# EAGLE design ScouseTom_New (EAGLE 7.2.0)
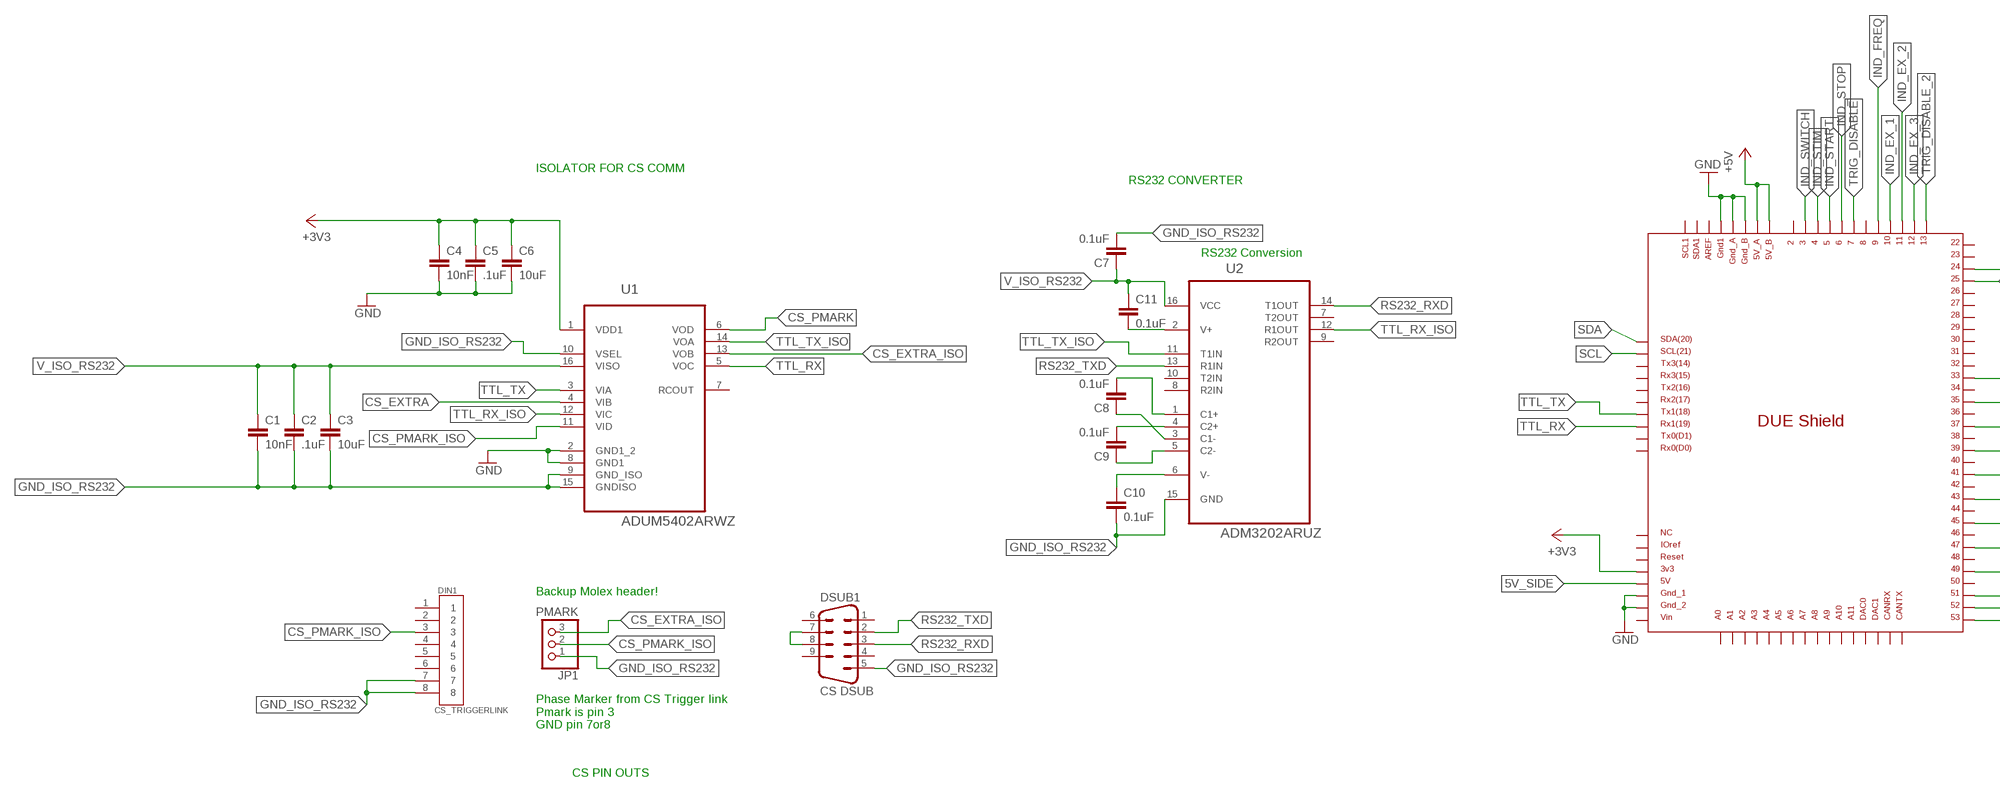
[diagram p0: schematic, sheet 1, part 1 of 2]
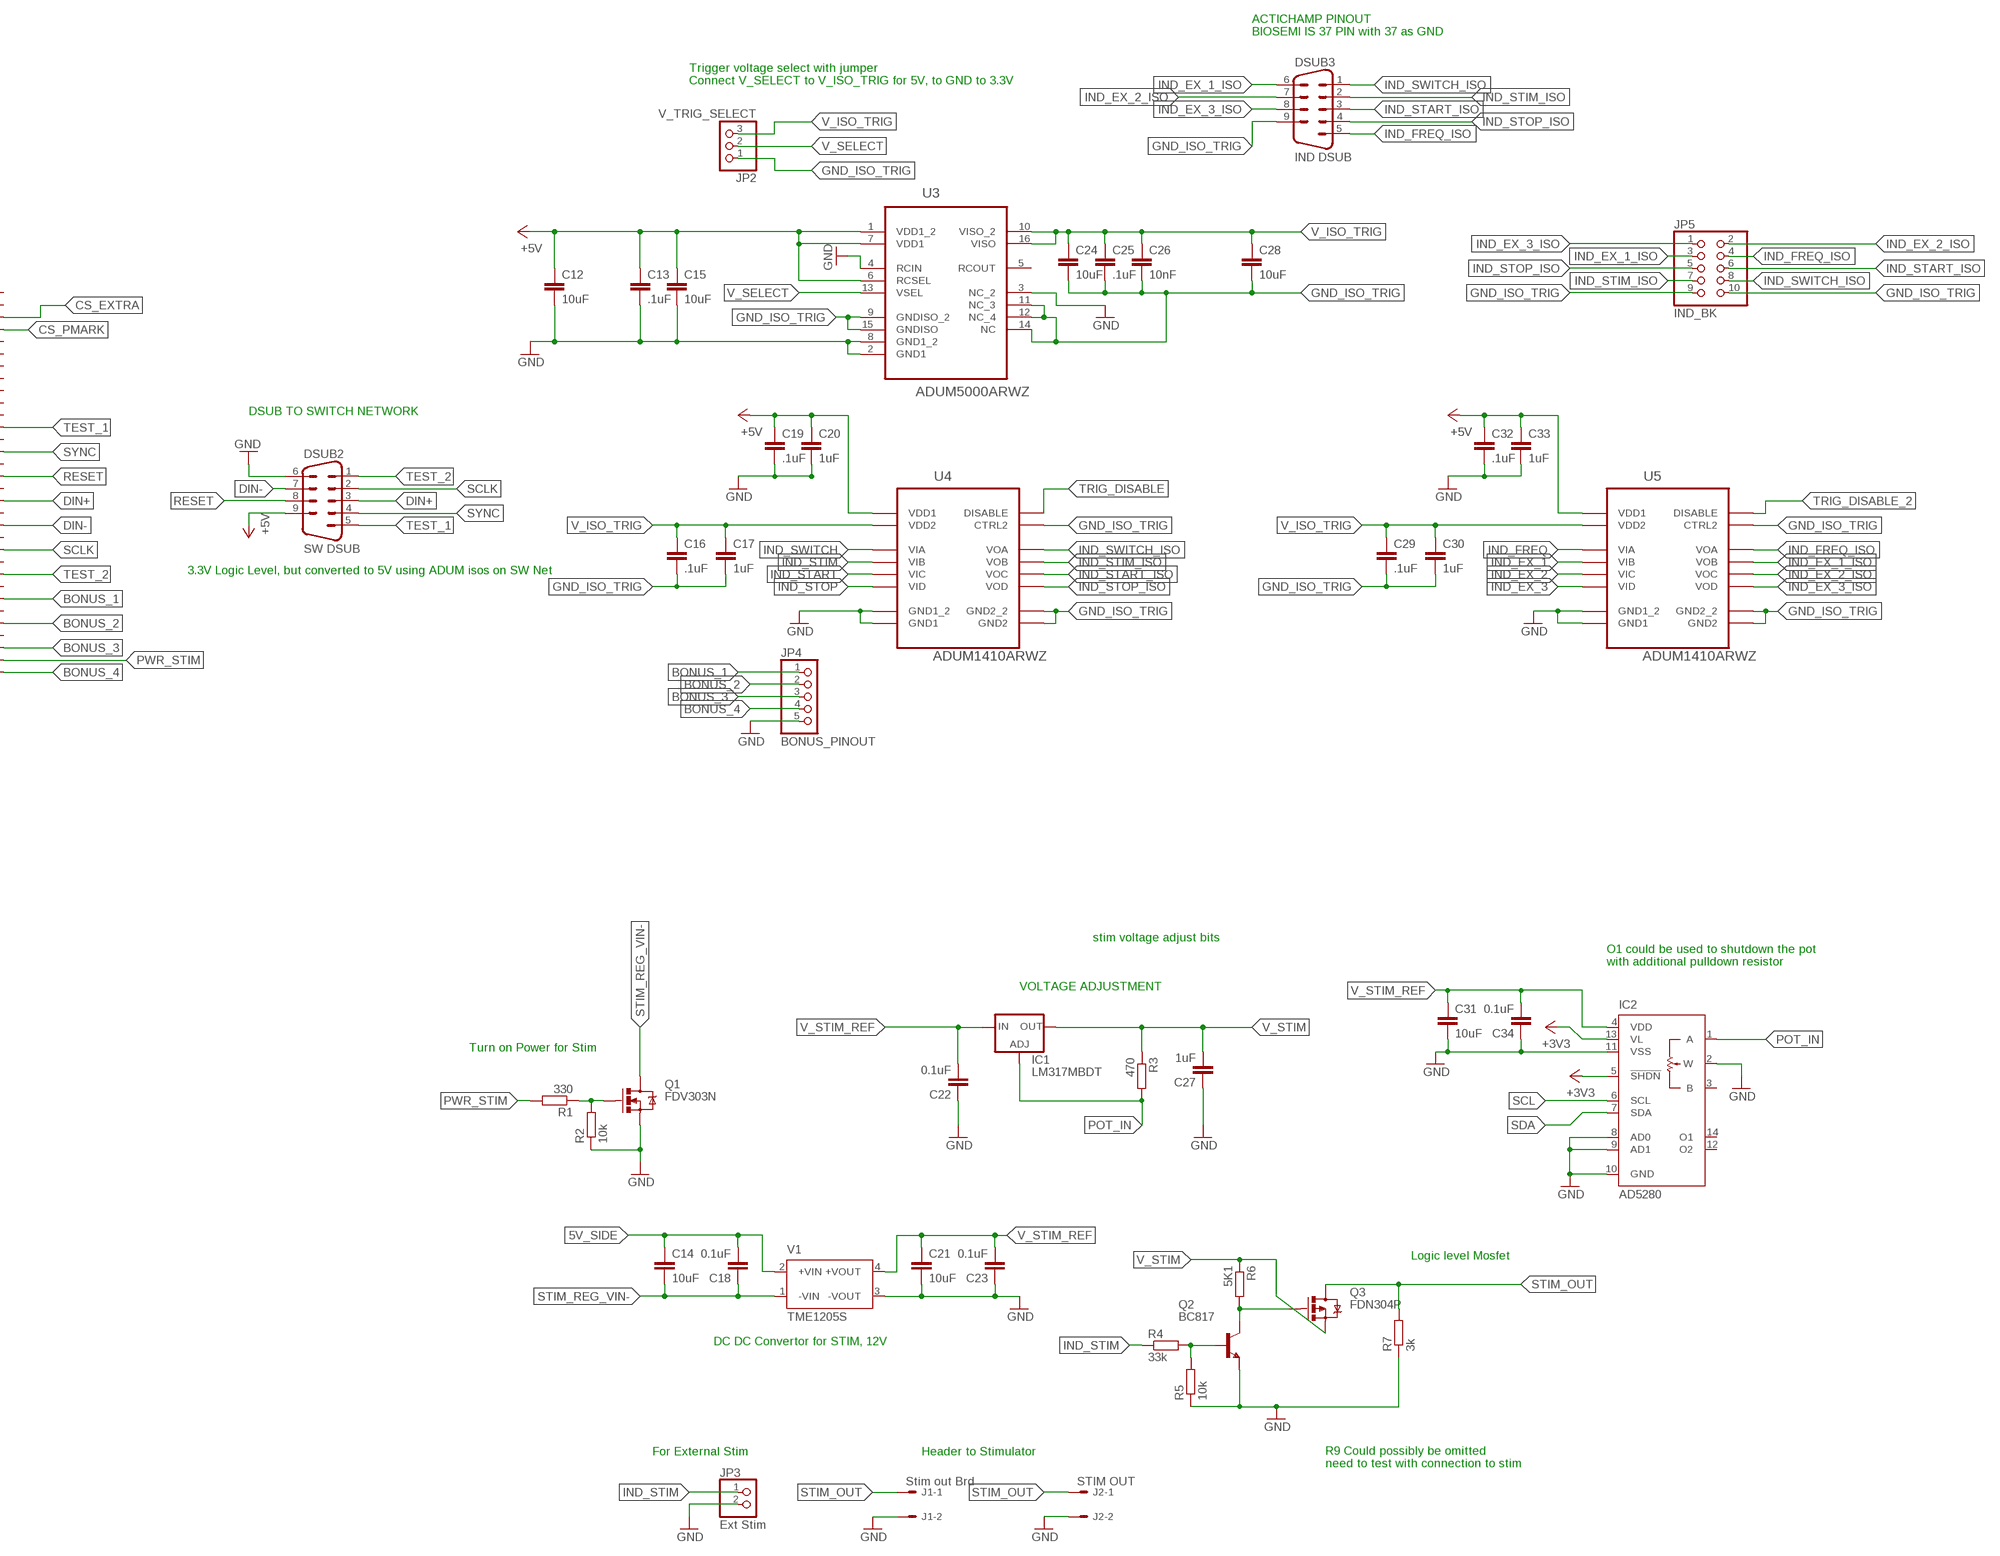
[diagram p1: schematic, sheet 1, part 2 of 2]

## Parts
ARD1  DUE(NOMID)  [DUE(NOMID)]
C1  10nF  C-EUC0805  [C0805]
C2  .1uF  C-EUC0805  [C0805]
C3  10uF  C-EUC0805  [C0805]
C4  10nF  C-EUC0805  [C0805]
C5  .1uF  C-EUC0805  [C0805]
C6  10uF  C-EUC0805  [C0805]
C7  0.1uF  C-EUC0805  [C0805]
C8  0.1uF  C-EUC0805  [C0805]
C9  0.1uF  C-EUC0805  [C0805]
C10  0.1uF  C-EUC0805  [C0805]
C11  0.1uF  C-EUC0805  [C0805]
C12  10uF  C-EUC0805  [C0805]
C13  .1uF  C-EUC0805  [C0805]
C14  10uF  C-EUC0805  [C0805]
C15  10uF  C-EUC0805  [C0805]
C16  .1uF  C-EUC0805  [C0805]
C17  1uF  C-EUC0805  [C0805]
C18  0.1uF  C-EUC0805  [C0805]
C19  .1uF  C-EUC0805  [C0805]
C20  1uF  C-EUC0805  [C0805]
C21  10uF  C-EUC0805  [C0805]
C22  0.1uF  C-EUC0805  [C0805]
C23  0.1uF  C-EUC0805  [C0805]
C24  10uF  C-EUC0805  [C0805]
C25  .1uF  C-EUC0805  [C0805]
C26  10nF  C-EUC0805  [C0805]
C27  1uF  C-EUC0805  [C0805]
C28  10uF  C-EUC0805  [C0805]
C29  .1uF  C-EUC0805  [C0805]
C30  1uF  C-EUC0805  [C0805]
C31  10uF  C-EUC0805  [C0805]
C32  .1uF  C-EUC0805  [C0805]
C33  1uF  C-EUC0805  [C0805]
C34  0.1uF  C-EUC0805  [C0805]
DIN1  CS_TRIGGERLINK  DIN8  [DIN8]
DSUB1  CS DSUB  DSUB9RA  [DSUB9]
DSUB2  SW DSUB  DSUB9RA  [DSUB9]
DSUB3  IND DSUB  DSUB9RA  [DSUB9]
IC1  LM317MBDT  [DPACK]
IC2  AD5280  [TSSOP14]
J1  Stim out Brd  22-27-2021-02  [6410-02]
J2  STIM OUT  22-05-7028-02  [7395-02]
JP1  PMARK  PINHD-1X3  [1X03]
JP2  V_TRIG_SELECT  PINHD-1X3  [1X03]
JP3  Ext Stim  PINHD-1X2  [1X02]
JP4  BONUS_PINOUT  PINHD-1X5  [1X05]
JP5  IND_BK  PINHD-2X5  [2X05]
Q1  FDV303N  MOSFET-NCHANNEL2N7002PW  [SOT323]
Q2  BC817  BC817-40SMD  [SOT23-BEC]
Q3  FDN304P  MOSFET-PCHANNEL  [SOT23-3]
R1  330  R-EU_R0805  [R0805]
R2  10k  R-EU_R0805  [R0805]
R3  470  R-EU_R0805  [R0805]
R4  33k  R-EU_R0805  [R0805]
R5  10k  R-EU_R0805  [R0805]
R6  5K1  R-EU_R0805  [R0805]
R7  3k  R-EU_R0805  [R0805]
U1  ADUM5402ARWZ  [SOIC127P1032X265-16N]
U2  ADM3202ARUZ  [SOP65P640X120-16N]
U3  ADUM5000ARWZ  [SOIC127P1032X265-16N]
U4  ADUM1410ARWZ  [SOIC127P1032X265-16N]
U5  ADUM1410ARWZ  [SOIC127P1032X265-16N]
V1  TME1205S  [TME]

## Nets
5V_SIDE: ARD1.5V C14.1 C18.2 V1.2(+VIN)
+3V3: ARD1.3V3 C4.1 C5.1 C6.1 IC2.5(!SHDN) IC2.13(VL) U1.1(VDD1)
+5V: ARD1.5V_A ARD1.5V_B C12.1 C13.1 C15.1 C19.1 C20.1 C32.1 C33.1 DSUB2.9 U3.1(VDD1_2) U3.6(RCSEL) U3.7(VDD1) U4.1(VDD1) U5.1(VDD1)
BONUS_1: ARD1.47 JP4.1
BONUS_2: ARD1.49 JP4.2
BONUS_3: ARD1.51 JP4.3
BONUS_4: ARD1.53 JP4.4
CS_EXTRA: ARD1.24 U1.4(VIB)
CS_EXTRA_ISO: JP1.3 U1.13(VOB)
CS_PMARK: ARD1.25 U1.6(VOD)
CS_PMARK_ISO: DIN1.3 JP1.2 U1.11(VID)
DIN+: ARD1.39 DSUB2.3
DIN-: ARD1.41 DSUB2.7
GND: ARD1.GND1 ARD1.GND_1 ARD1.GND_2 ARD1.GND_A ARD1.GND_B C4.2 C5.2 C6.2 C12.2 C13.2 C15.2 C19.2 C20.2 C21.2 C22.1 C23.1 C27.1 C31.2 C32.2 C33.2 C34.1 DSUB2.6 IC2.2(W) IC2.8(AD0) IC2.9(AD1) IC2.10(GND) IC2.11(VSS) J1.2 J2.2 JP3.2 JP4.5 Q1.2(S) Q2.E R2.1 R5.1 R7.1 U1.2(GND1_2) U1.8(GND1) U3.2(GND1) U3.3(NC_2) U3.4(RCIN) U3.8(GND1_2) U4.2(GND1_2) U4.8(GND1) U5.2(GND1_2) U5.8(GND1) V1.3(-VOUT)
GND_ISO_RS232: C1.2 C2.2 C3.2 C7.2 C10.2 DIN1.7 DIN1.8 DSUB1.5 JP1.1 U1.9(GND_ISO) U1.10(VSEL) U1.15(GNDISO) U2.15(GND)
GND_ISO_TRIG: C16.2 C17.2 C24.2 C25.2 C26.2 C28.2 C29.2 C30.2 DSUB3.9 JP2.1 JP5.9 JP5.10 U3.9(GNDISO_2) U3.11(NC_3) U3.12(NC_4) U3.14(NC) U3.15(GNDISO) U4.9(GND2_2) U4.10(CTRL2) U4.15(GND2) U5.9(GND2_2) U5.10(CTRL2) U5.15(GND2)
IND_EX_1: ARD1.10 U5.4(VIB)
IND_EX_1_ISO: DSUB3.6 JP5.3 U5.13(VOB)
IND_EX_2: ARD1.11 U5.5(VIC)
IND_EX_2_ISO: DSUB3.7 JP5.2 U5.12(VOC)
IND_EX_3: ARD1.12 U5.6(VID)
IND_EX_3_ISO: DSUB3.8 JP5.1 U5.11(VOD)
IND_FREQ: ARD1.9 U5.3(VIA)
IND_FREQ_ISO: DSUB3.5 JP5.4 U5.14(VOA)
IND_START: ARD1.5 U4.5(VIC)
IND_START_ISO: DSUB3.3 JP5.6 U4.12(VOC)
IND_STIM: ARD1.4 JP3.1 R4.1 U4.4(VIB)
IND_STIM_ISO: DSUB3.2 JP5.7 U4.13(VOB)
IND_STOP: ARD1.6 U4.6(VID)
IND_STOP_ISO: DSUB3.4 JP5.5 U4.11(VOD)
IND_SWITCH: ARD1.3 U4.3(VIA)
IND_SWITCH_ISO: DSUB3.1 JP5.8 U4.14(VOA)
N$1: Q2.B R4.2 R5.2
N$3: Q2.C Q3.1(G) R6.2
N$4: DSUB1.7 DSUB1.8
N$5: Q1.1(G) R1.1 R2.2
N$22: C8.2 U2.1(C1+)
N$23: C8.1 U2.3(C1-)
N$24: C9.2 U2.4(C2+)
N$25: C9.1 U2.5(C2-)
N$26: C11.2 U2.2(V+)
N$27: C10.1 U2.6(V-)
POT_IN: IC1.1(ADJ) IC2.1(A) R3.2
PWR_STIM: ARD1.52 R1.2
RESET: ARD1.37 DSUB2.8
RS232_RXD: DSUB1.3 U2.14(T1OUT)
RS232_TXD: DSUB1.2 U2.13(R1IN)
SCL: ARD1.SCL IC2.6(SCL)
SCLK: ARD1.43 DSUB2.2
SDA: ARD1.SDA IC2.7(SDA)
STIM_OUT: J1.1 J2.1 Q3.3(D) R7.2
STIM_REG_VIN-: C14.2 C18.1 Q1.3(D) V1.1(-VIN)
SYNC: ARD1.35 DSUB2.4
TEST_1: ARD1.33 DSUB2.5
TEST_2: ARD1.45 DSUB2.1
TRIG_DISABLE: ARD1.7 U4.7(DISABLE)
TRIG_DISABLE_2: ARD1.13 U5.7(DISABLE)
TTL_RX: ARD1.RX1 U1.5(VOC)
TTL_RX_ISO: U1.12(VIC) U2.12(R1OUT)
TTL_TX: ARD1.TX1 U1.3(VIA)
TTL_TX_ISO: U1.14(VOA) U2.11(T1IN)
V_ISO_RS232: C1.1 C2.1 C3.1 C7.1 C11.1 U1.16(VISO) U2.16(VCC)
V_ISO_TRIG: C16.1 C17.1 C24.1 C25.1 C26.1 C28.1 C29.1 C30.1 JP2.3 U3.10(VISO_2) U3.16(VISO) U4.16(VDD2) U5.16(VDD2)
V_SELECT: JP2.2 U3.13(VSEL)
V_STIM: C27.2 IC1.4(OUT) Q3.2(S) R3.1 R6.1
V_STIM_REF: C21.1 C22.2 C23.2 C31.1 C34.2 IC1.3(IN) IC2.4(VDD) V1.4(+VOUT)
Unconnected: ARD1.2 ARD1.8 ARD1.22 ARD1.23 ARD1.26 ARD1.27 ARD1.28 ARD1.29 ARD1.30 ARD1.31 ARD1.32 ARD1.34 ARD1.36 ARD1.38 ARD1.40 ARD1.42 ARD1.44 ARD1.46 ARD1.48 ARD1.50 ARD1.A0 ARD1.A1 ARD1.A2 ARD1.A3 ARD1.A4 ARD1.A5 ARD1.A6 ARD1.A7 ARD1.A8 ARD1.A9 ARD1.A10 ARD1.A11 ARD1.AREF ARD1.CANRX ARD1.CANTX ARD1.DAC0 ARD1.DAC1 ARD1.IOREF ARD1.NC ARD1.RESET ARD1.RX0 ARD1.RX2 ARD1.RX3 ARD1.SCL1 ARD1.SDA1 ARD1.TX0 ARD1.TX2 ARD1.TX3 ARD1.VIN DIN1.1 DIN1.2 DIN1.4 DIN1.5 DIN1.6 DSUB1.1 DSUB1.4 DSUB1.6 DSUB1.9 IC2.3(B) IC2.12(O2) IC2.14(O1) U1.7(RCOUT) U2.7(T2OUT) U2.8(R2IN) U2.9(R2OUT) U2.10(T2IN) U3.5(RCOUT)

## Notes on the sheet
- ACTICHAMP PINOUT
  BIOSEMI IS 37 PIN with 37 as GND
- Trigger voltage select with jumper
  Connect V_SELECT to V_ISO_TRIG for 5V, to GND to 3.3V
- ISOLATOR FOR CS COMM
- RS232 CONVERTER
- RS232 Conversion
- DSUB TO SWITCH NETWORK
- 3.3V Logic Level, but converted to 5V using ADUM isos on SW Net
- Backup Molex header!
- Phase Marker from CS Trigger link
  Pmark is pin 3
  GND pin 7or8
- CS PIN OUTS
- stim voltage adjust bits
- O1 could be used to shutdown the pot
  with additional pulldown resistor
- VOLTAGE ADJUSTMENT
- Turn on Power for Stim
- Logic level Mosfet
- DC DC Convertor for STIM, 12V
- For External Stim | Header to Stimulator
- R9 Could possibly be omitted
  need to test with connection to stim

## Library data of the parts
ARD1 = DUElib130425_JAMES:DUE(NOMID)
C1-C34 = resistor:C-EU: CAPACITOR, European symbol
DIN1 = mini din 8 james:DIN8
DSUB1-DSUB3 = DSUBJAMES:DSUB9RA
IC1 = v-reg:LM317?*: 500 mA Adjustable Output Positive Voltage Regulator Source: http://www.onsemi.co.jp .. LM317M-D.PDF
IC2 = analog-devices:AD5280: Single +15 V/±5 V, 256-Position, I2C-Compatible Digital Potentiometer Source: http://www.analog.com/static/imported-files/data_sheets/AD5280_5282.pdf; MF: ALTERA CORPORATION; MPN: AD5280BRUZ20; OC_FARNELL: 1464325; OC_NEWARK: 59K3840
J1 = con-molex:22-?-02: CONNECTOR; OC_FARNELL: unknown; OC_NEWARK: unknown
J2 = con-molex:22-?-02: CONNECTOR; OC_FARNELL: 9731601; OC_NEWARK: unknown
JP1 JP2 = pinhead:PINHD-1X3: PIN HEADER
JP3 = pinhead:PINHD-1X2: PIN HEADER
JP4 = pinhead:PINHD-1X5: PIN HEADER
JP5 = pinhead:PINHD-2X5: PIN HEADER
Q1 = SparkFun-DiscreteSemi:MOSFET-NCHANNEL: Common NMOSFET Parts MFG P/NStore IDProd ID FDD8780TRANS-09984 SI7820DNTRANS-11055 FDS6630AIC-08089 2N7002PWTRANS-11151 FQP30N06L COM-10213TRANS-10060 BSS123LT1GTRANS-08345 BSS138TRANS-00830 BS170 2N7000; PROD_ID: TRANS-11151
Q2 = transistor-npn:BC817*: NPN Transistor
Q3 = SparkFun-DiscreteSemi:MOSFET-PCHANNEL: Generic PMOSFET IRLML2244 - TRANS-11153 (SOT-23 -20V -4.3A) (1.Gate 2.Source 3.Drain) FQP27P06 - COM-10349 (TO-220 -60V -27A) (1.Gate 2.Source 3.Drain); PROD_ID: TRANS-08285
R1-R7 = resistor:R-EU_: RESISTOR, European symbol
U1 = Analog Devices_By_element14_Batch_1:ADUM5402ARWZ: Quad-Channel Isolators with Integrated DC-to-DC Converter; MPN: ADUM5402ARWZ; OC_FARNELL: 1838922; OC_NEWARK: 11N8824; PACKAGE: SOIC-16; SUPPLIER: Analog Devices
U2 = Analog Devices_By_element14_Batch_1:ADM3202ARUZ: Low Power, 3.3 V, RS-232 Line Drivers/Receivers; MPN: ADM3202ARUZ; OC_FARNELL: 9425586; OC_NEWARK: 59K2064; PACKAGE: TSSOP-16; SUPPLIER: Analog Devices
U3 = Analog Devices_By_element14_Batch_1:ADUM5000ARWZ: 2.5 kV, Isolated DC-to-DC Converter; MPN: ADUM5000ARWZ; OC_FARNELL: 1701256; OC_NEWARK: 19P8235; PACKAGE: SOIC-16; SUPPLIER: Analog Devices
U4 U5 = ADI-Phase-2:ADUM1410ARWZ: ISOLATOR, DGTL, 4CHAN; MPN: ADUM1410ARWZ; OC_FARNELL: 2067770; OC_NEWARK: 73T8174; PACKAGE: 16-Lead SOIC_W; SUPPLIER: Analog Devices
V1 = traco-electronic:TME?*: DC/DC Converter TME Series 1 Watt Source: www.tracopower.com .. tme.pdf; MPN: TME 1205S; OC_FARNELL: 1007542; OC_NEWARK: 51R5325

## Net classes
1 power: width 0.61 mm, drill 0.61 mm, clearance 0.254 mm
2 gnd: width 0.305 mm, drill 0.559 mm, clearance 0.254 mm
3 usbvcc: width 0.508 mm, drill 0.61 mm, clearance 0.254 mm
4 aref: width 0.406 mm, drill 0.61 mm, clearance 0.254 mm

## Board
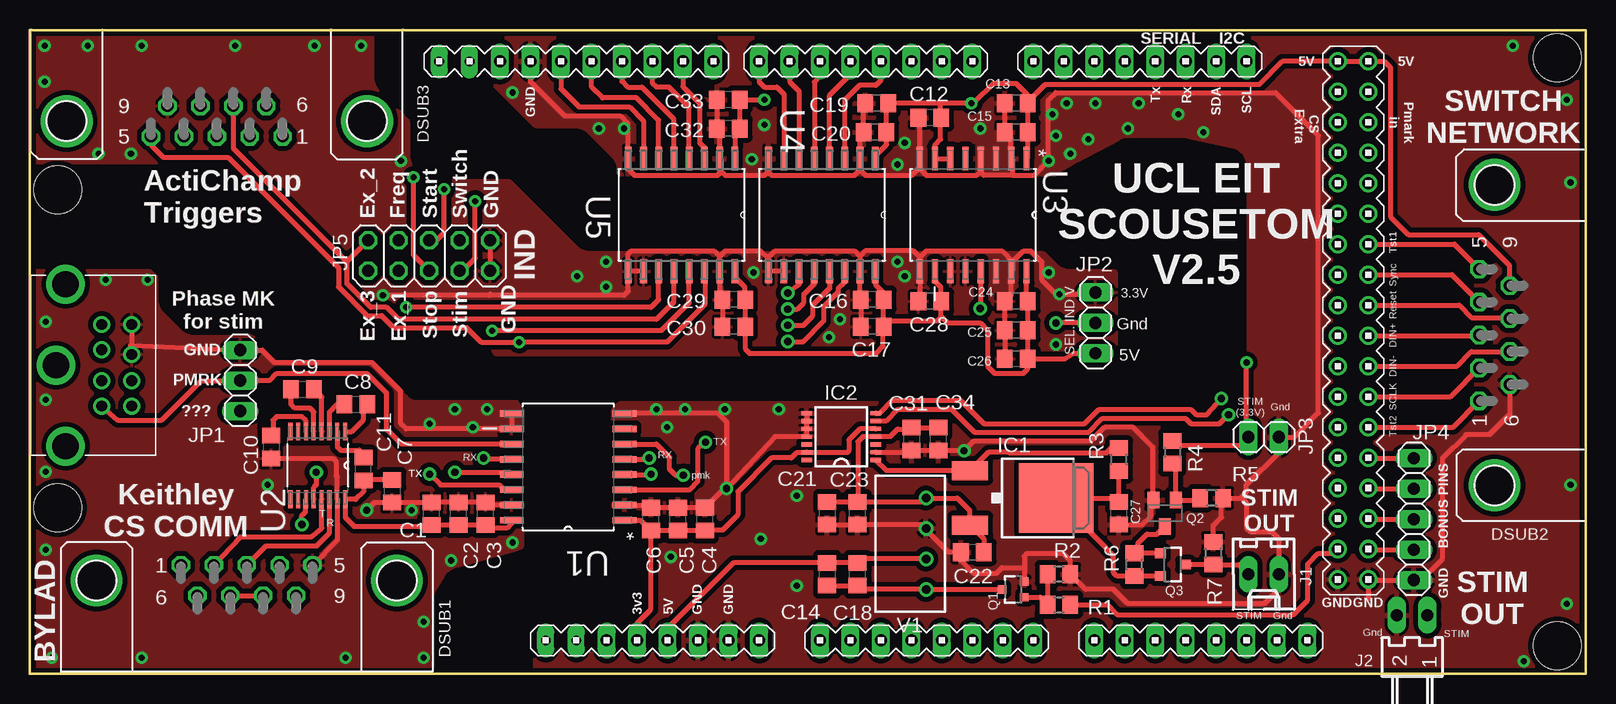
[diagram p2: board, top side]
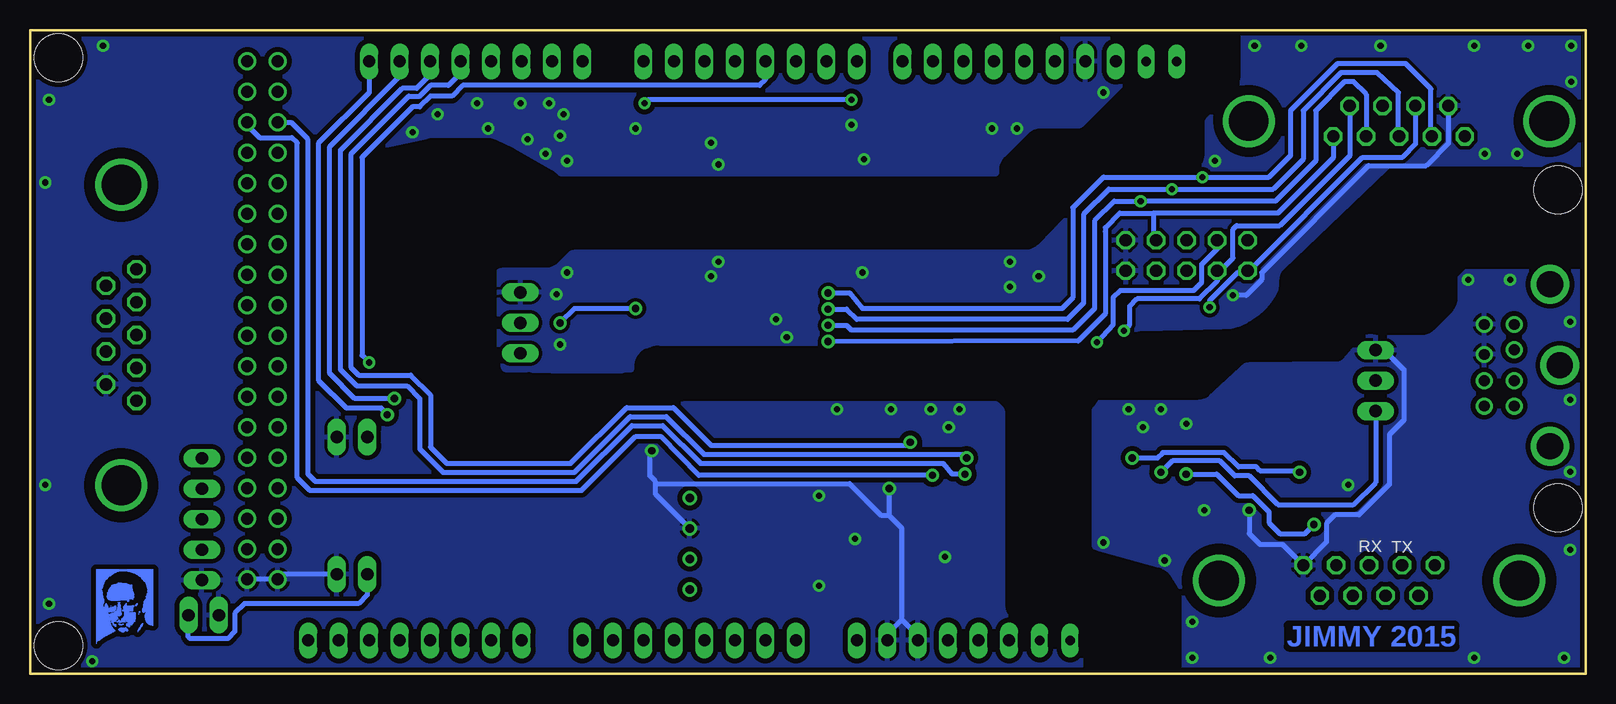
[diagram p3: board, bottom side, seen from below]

Size 129.69 x 53.67 mm. Coordinates in mm from the lower left corner, seen from the top.
Outline: 129.69,53.67 0,53.67 0,0 129.69,0 129.69,53.67
Copper layers (1*16): Top 0.035mm / dielectric 1.5mm / Bottom 0.035mm
Design rules "pcbtrain": minimum track width 0.2mm, minimum drill 0.4mm, track to track 0.2mm, track to pad 0.2mm, pad to pad 0.2mm, via to via 0.2mm, smd to smd 0mil, copper to edge 10mil, drill to drill 0.2mm, minimum pad ring 10mil, minimum via ring 10mil, stop-mask expansion 0.125mm, vias tented up to drill 0mil, thermal gap 10mil
Holes 4 mm at 127.31,51.36 127.31,2.36 2.31,13.86 2.31,40.36
tRestrict: area -5.2,-2.6 to 100.8,56.4
bRestrict: area -5.2,-2.6 to 100.8,56.4

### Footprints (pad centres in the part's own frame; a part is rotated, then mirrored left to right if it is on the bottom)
DUE(NOMID) = drill 1 long: 2 -5.08,25.4; 3 -7.62,25.4; 3V3 -27.94,-22.86; 4 -10.16,25.4; 5 -12.7,25.4; 5V -25.4,-22.86; 6 -15.24,25.4; 7 -17.78,25.4; 8 -21.59,25.4; 9 -24.13,25.4; 10 -26.67,25.4; 11 -29.21,25.4; 12 -31.75,25.4; 13 -34.29,25.4; A0 -12.7,-22.86; A1 -10.16,-22.86; A2 -7.62,-22.86; A3 -5.08,-22.86; A4 -2.54,-22.86; A5 0,-22.86; A6 2.54,-22.86; A7 5.08,-22.86; A8 10.16,-22.86; A9 12.7,-22.86; A10 15.24,-22.86; A11 17.78,-22.86; AREF -39.37,25.4; CANRX 25.4,-22.86; CANTX 27.94,-22.86; DAC0 20.32,-22.86; DAC1 22.86,-22.86; GND1 -36.83,25.4; GND_1 -22.86,-22.86; GND_2 -20.32,-22.86; RESET -30.48,-22.86; RX0 0,25.4; RX1 17.78,25.4; RX2 12.7,25.4; RX3 7.62,25.4; SCL 22.86,25.4; SDA 20.32,25.4; TX0 -2.54,25.4; TX1 15.24,25.4; TX2 10.16,25.4; TX3 5.08,25.4; VIN -17.78,-22.86 | drill 1: 5V_A 30.48,25.4; 5V_B 33.02,25.4; 22 30.48,22.86; 23 33.02,22.86; 24 30.48,20.32; 25 33.02,20.32; 26 30.48,17.78; 27 33.02,17.78; 28 30.48,15.24; 29 33.02,15.24; 30 30.48,12.7; 31 33.02,12.7; 32 30.48,10.16; 33 33.02,10.16; 34 30.48,7.62; 35 33.02,7.62; 36 30.48,5.08; 37 33.02,5.08; 38 30.48,2.54; 39 33.02,2.54; 40 30.48,0; 41 33.02,0; 42 30.48,-2.54; 43 33.02,-2.54; 44 30.48,-5.08; 45 33.02,-5.08; 46 30.48,-7.62; 47 33.02,-7.62; 48 30.48,-10.16; 49 33.02,-10.16; 50 30.48,-12.7; 51 33.02,-12.7; 52 30.48,-15.24; 53 33.02,-15.24; GND_A 30.48,-17.78; GND_B 33.02,-17.78 | drill 0.8 pad 1.422 long: IOREF -33.02,-22.86; NC -35.56,-22.86; SCL1 -44.45,25.4; SDA1 -41.91,25.4
C0805 = smd 1.3 x 1.5: 1 -0.95,0; 2 0.95,0
DIN8 = drill 0.9: 1 -1.3,-3.8; 2 1.3,-3.8; 3 -3.4,-3.8; 4 -1.3,-6.3; 5 3.4,-3.8; 6 -3.4,-6.3; 7 0.9,-6.3; 8 3.4,-6.3 | drill 2.2: P$1 0,0; P$2 -6.75,-0.8; P$3 6.75,-0.8
DSUB9 = drill 1.016 octagon: 1 -5.486,0; 2 -2.743,0; 3 0,0; 4 2.743,0; 5 5.486,0; 6 -4.115,-2.54; 7 -1.372,-2.54; 8 1.372,-2.54; 9 4.115,-2.54 | drill 3.302: 10 -12.522,-1.27; 11 12.522,-1.27
DPACK = smd 1.6 x 3: 1 -2.28,-4.8; 3 2.28,-4.8 | smd 5.8 x 6.2: 4 0,2.38
TSSOP14 = smd 0.9 x 0.35: 1 -2.875,1.95; 2 -2.875,1.3; 3 -2.875,0.65; 4 -2.875,0; 5 -2.875,-0.65; 6 -2.875,-1.3; 7 -2.875,-1.95; 8 2.875,-1.95; 9 2.875,-1.3; 10 2.875,-0.65; 11 2.875,0; 12 2.875,0.65; 13 2.875,1.3; 14 2.875,1.95
6410-02 = drill 1.016 long: 1 1.27,0; 2 -1.27,0
7395-02 = drill 1.016 long: 1 1.27,0; 2 -1.27,0
1X03 = drill 1.016 long: 1 -2.54,0; 2 0,0; 3 2.54,0
1X02 = drill 1.016 long: 1 -1.27,0; 2 1.27,0
1X05 = drill 1.016 long: 1 -5.08,0; 2 -2.54,0; 3 0,0; 4 2.54,0; 5 5.08,0
2X05 = drill 1.016 octagon: 1 -5.08,-1.27; 2 -5.08,1.27; 3 -2.54,-1.27; 4 -2.54,1.27; 5 0,-1.27; 6 0,1.27; 7 2.54,-1.27; 8 2.54,1.27; 9 5.08,-1.27; 10 5.08,1.27
SOT323 = smd 0.7 x 0.7: 1 -0.65,-0.925; 2 0.65,-0.925; 3 0,0.925
SOT23-BEC = smd 1 x 1.4: B -0.95,-1.1; C 0,1.1; E 0.95,-1.1
SOT23-3 = smd 0.8 x 0.9: 1 -0.95,-1; 2 0.95,-1; 3 0,1.1
R0805 = smd 1.3 x 1.5: 1 -0.95,0; 2 0.95,0
SOIC127P1032X265-16N = smd 1.981 x 0.533: 1 -4.699,4.445; 2 -4.699,3.175; 3 -4.699,1.905; 4 -4.699,0.635; 5 -4.699,-0.635; 6 -4.699,-1.905; 7 -4.699,-3.175; 8 -4.699,-4.445; 9 4.699,-4.445; 10 4.699,-3.175; 11 4.699,-1.905; 12 4.699,-0.635; 13 4.699,0.635; 14 4.699,1.905; 15 4.699,3.175; 16 4.699,4.445
SOP65P640X120-16N = smd 1.473 x 0.356: 1 -2.819,2.286; 2 -2.819,1.626; 3 -2.819,0.965; 4 -2.819,0.33; 5 -2.819,-0.33; 6 -2.819,-0.965; 7 -2.819,-1.626; 8 -2.819,-2.286; 9 2.819,-2.286; 10 2.819,-1.626; 11 2.819,-0.965; 12 2.819,-0.33; 13 2.819,0.33; 14 2.819,0.965; 15 2.819,1.626; 16 2.819,2.286
SOIC127P1032X265-16N' = smd 1.981 x 0.559: 1 -4.699,4.445; 2 -4.699,3.175; 3 -4.699,1.905; 4 -4.699,0.635; 5 -4.699,-0.635; 6 -4.699,-1.905; 7 -4.699,-3.175; 8 -4.699,-4.445; 9 4.699,-4.445; 10 4.699,-3.175; 11 4.699,-1.905; 12 4.699,-0.635; 13 4.699,0.635; 14 4.699,1.905; 15 4.699,3.175; 16 4.699,4.445
TME = drill 0.7 pad 1.1: 1 -3.81,0; 2 -1.27,0; 3 1.27,0; 4 3.81,0

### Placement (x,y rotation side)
ARD1  78.56,25.65 0 top
C1  33.46,13.36 90 top
C2  35.71,13.36 90 top
C3  37.96,13.36 90 top
C4  56.27,12.91 90 top
C5  54.02,12.91 90 top
C6  51.77,12.91 90 top
C7  30.2,15.23 270 top
C8  27.16,22.46 0 top
C9  22.71,23.74 0 top
C10  20.09,18.91 270 top
C11  27.8,17.09 90 top
C12  75.02,46.36 180 top
C13  82.22,47.56 180 top
C14  66.44,8.32 270 top
C15  82.22,45.16 180 top
C16  70.22,31.21 180 top
C17  70.22,28.96 180 top
C18  68.98,8.32 90 top
C19  70.59,47.56 180 top
C20  70.44,45.16 180 top
C21  66.44,13.39 270 top
C22  78.55,10.16 0 top
C23  68.98,13.39 90 top
C24  82.22,31.06 180 top
C25  82.22,28.65 180 top
C26  82.22,26.25 180 top
C27  90.78,13.39 90 top
C28  75.02,31.06 180 top
C29  58.66,31.21 180 top
C30  58.66,28.96 180 top
C31  73.48,19.58 270 top
C32  58.21,45.45 180 top
C33  58.21,47.86 180 top
C34  75.72,19.58 90 top
DIN1  2.17,25.72 90 top
DSUB1  18.06,9.07 0 top
DSUB2  120.81,28.25 90 top
DSUB3  15.57,44.8 180 top
IC1  83.16,14.66 270 top
IC2  67.62,19.78 180 top
J1  102.84,8.32 180 top
J2  115.22,4.91 0 top
JP1  17.52,24.46 270 top
JP2  88.81,29.25 270 top
JP3  102.84,19.75 0 top
JP4  115.36,12.91 270 top
JP5  33.27,34.87 0 top
Q1  81.96,7.05 90 top
Q2  94.59,13.39 180 top
Q3  95.22,9.12 270 top
R1  85.77,5.78 0 top
R2  85.77,8.32 180 top
R3  90.78,17.88 90 top
R4  95.22,18.47 270 top
R5  98.5,14.66 180 top
R6  92.05,9.12 90 top
R7  98.63,10.07 270 top
U1  44.87,17.25 180 top
U2  23.98,17.39 270 top
U3  78.61,38.25 270 top
U4  ADUM1410ARWZ  [SOIC127P1032X265-16N']  66.02,38.25 270 top
U5  ADUM1410ARWZ  [SOIC127P1032X265-16N']  54.31,38.25 270 top
V1  74.7,10.86 90 top

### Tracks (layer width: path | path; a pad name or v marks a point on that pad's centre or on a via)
5V_SIDE
  Top 0.406: V1.2 69.3,9.59 C18.2 C14.1 58.62,9.27 53.16,3.8 ARD1.5V
+3V3
  Top 0.406: C6.1 C5.1 C4.1 56.77,12 57.77,12 59.02,13.25 59.02,15.21 61.81,18 63.46,18 63.91,18.46 64.72,18.46 IC2.13 64.77,18.46 68.11,18.46 68.27,18.61 68.27,19.5 69.19,20.43 IC2.5 | C6.1 51.77,5.39 50.61,4.25 ARD1.3V3 | U1.1 50.91,12.81 C6.1
+5V  (via drill 0.51)
  Top 0.406: U3.1 83.16,43.06 C15.1 C13.1 83.16,47.75 | U4.1 70.56,43.06 70.56,43.25 71.42,44.11 71.42,45.12 C20.1 71.39,47.41 C19.1 75.92,47.56 | U3.6 U3.7 75.44,44.08 75.92,44.56 75.92,46.31 C12.1 75.92,46.41 75.92,47.56 | 75.92,47.56 v78.47,47.56 78.67,47.56 80.31,49.2 82.22,49.2 83.16,48.25 83.16,47.75 | U5.1 58.76,45.05 C32.1 C33.1 v61.21,47.86 | DSUB2.9 123.31,32.4 123.31,34.06 120.77,36.61 114.91,36.61 113.41,38.11 113.41,50.56 112.91,51.06 ARD1.5V_B ARD1.5V_A 104.41,51.06 102.47,49.11 84.61,49.11 83.27,47.75 83.16,47.75
  Bottom 0.406: v61.21,47.86 78.17,47.86 v78.47,47.56
BONUS_1
  Top 0.406: ARD1.47 111.62,17.98 JP4.1
BONUS_2
  Top 0.406: ARD1.49 111.62,15.45 JP4.2
BONUS_3
  Top 0.406: ARD1.51 111.62,12.91 JP4.3
BONUS_4
  Top 0.406: ARD1.53 111.62,10.37 JP4.4
CS_EXTRA  (via drill 0.6)
  Top 0.406: U1.4 51.73,16.62 v51.77,16.66
  Bottom 0.406: ARD1.24 107.94,45.97 106.52,44.56 106.52,16.66 105.91,16.05 84.16,16.05 79.52,20.71 76.97,20.71 73.81,17.55 53.56,17.55 52.81,16.66 v51.77,16.66
CS_EXTRA_ISO  (via drill 0.6)
  Top 0.406: v35.41,16.8 39.98,16.8 U1.13
  Bottom 0.406: JP1.3 17.52,15.95 19.36,14.11 25.66,14.11 28.06,16.5 29.27,16.5 30.52,17.75 34.46,17.75 v35.41,16.8
CS_PMARK  (via drill 0.6)
  Top 0.406: U1.6 52.21,19.16 53.31,18.05 53.31,17.05 53.81,16.55 v54.46,16.55
  Bottom 0.406: ARD1.25 111.58,45.72 110.56,44.7 107.86,44.7 107.41,44.25 107.41,16.36 106.36,15.3 83.72,15.3 79.22,19.81 77.11,19.81 73.97,16.55 v54.46,16.55
CS_PMARK_ISO
  Top 0.406: DIN1.3 7.29,21.15 10.96,21.15 14.26,24.46 JP1.2 19.96,24.46 20.56,25.06 28.06,25.06 29.71,23.4 29.71,20.4 30.96,19.16 U1.11
DIN+
  Top 0.406: ARD1.39 120.77,28.2 DSUB2.3
DIN-
  Top 0.406: ARD1.41 118.97,25.65 120.16,26.86 123.34,26.86 DSUB2.7
GND  (via drill 0.51, 0.6)
  Top 0.406: R7.1 98.63,12.37 99.31,13.05 99.31,14.53 R5.1 101,14.66 | 101,14.66 101.41,14.25 101.41,12.16 101.72,11.86 103.52,11.86 104.11,11.25 J1.2 104.11,7.05 102.91,5.86 91.52,5.86 90.31,7.05 87.98,7.05 R2.1 86.72,9.45 86.11,10.05 83.11,10.05 82.88,9.82 82.88,8.86 | 101,14.66 101,14.75 101.41,15.16 101.41,15.75 104.11,18.46 | C13.2 C15.2 81.79,44.63 U3.2 81.91,42.83 81.91,41.7 | 69.19,44.63 C20.2 | C12.2 74.17,46.25 U3.8 74.17,42.16 | 74.17,42.16 74.17,42.1 74.72,41.56 78.92,41.56 79.22,41.86 | 79.22,41.86 79.22,42.92 U3.4 | IC2.8 64.81,21.66 64.81,21.15 IC2.9 IC2.10 IC2.11 62.09,19.78 v58.06,15.46 | U1.8 48.86,21.7 48.91,21.75 57.31,21.75 58.06,21 v58.06,15.46 | C21.2 C23.1 74.38,12.45 V1.3 74.7,12.03 76.52,10.21 77.56,10.21 C22.1 77.6,9.42 78.61,8.41 80.56,8.41 81.02,8.86 82.88,8.86 | C21.2 66.76,12.12 | U5.2 57.49,42.03 57.96,41.56 61.21,41.56 61.57,41.91 | 61.52,42.9 U4.8 61.57,41.91 | 69.19,42.03 U4.2 69.19,44.86 C20.2 | 69.19,42.03 69.67,41.56 73.52,41.56 74.11,42.16 74.17,42.16 | 81.91,41.7 81.91,41.56 79.52,41.56 79.22,41.86 | 69.19,42.03 68.72,41.56 61.81,41.56 61.57,41.8 61.57,41.91 | U5.2 57.61,42.83 57.61,41.86 57.31,41.56 50.41,41.56 49.81,42.16 49.81,42.9 U5.8 49.81,43.01 49.81,45.91 49.21,46.5 44.56,46.5 41.73,49.34 ARD1.GND1 | C33.2 C32.2 57.49,45.23 U5.2 | 48.79,14.08 U1.2 51.54,14.08 C6.2 C5.2 C4.2 58.06,15.66 v58.06,15.46 | C21.2 | IC2.2 73.34,18.48 C31.2 C34.1 75.75,18.61 v77.86,18.61 78.67,19.4 88.41,19.4 89.56,20.56 91.97,20.56 93.61,18.9 93.61,14.47 Q2.E 93.47,14.32 93.47,13.21 92.7,12.45 C27.1 | 82.88,8.86 Q1.2 | 81.91,41.7 82.06,41.56 83.72,41.56 v84.91,42.75 84.91,47.86 85.52,48.45 103.81,48.45 107.41,44.86 107.41,21.75 105.41,19.75 JP3.2
  Top 0.406: DSUB2.6 123.36,21.64 121.66,19.96 119.72,19.96 117.77,18 117.77,9.61 115.98,7.82 JP4.5 111.62,7.82 ARD1.GND_B 111.61,7.84 111.61,6.3 | C20.2 69.48,47.41 C19.2
  Bottom 0.406: ARD1.GND_B ARD1.GND_A 108.59,8.32 J1.2 | ARD1.GND_1 55.7,3.18 57.02,4.5 | ARD1.GND_2 58.23,3.29 57.02,4.5 | v77.86,18.61 78.02,18.46 78.02,16.5 77.56,16.05 77.56,15 V1.3 | 57.02,4.5 57.02,12.16 58.06,13.21 | 58.06,13.21 v58.06,15.46 | 58.06,13.21 58.71,13.21 61.36,15.86 77.56,15.86
  other vias: 52.21,22.06 53.11,20.56 54.61,22.06 85.22,46.66 79.22,45.45 72.31,42.45 72.92,44.25 49.52,45.45 47.41,45.45 60.16,42.91 61.21,45.75 86.41,47.56 40.21,48.45 88.81,47.56 92.41,47.56 95.72,46.66 97.81,45.16 91.52,45.45 88.22,44.56 86.72,43.36 85.52,44.86 62.41,22.06 57.91,22.06 63.91,14.86 60.91,11.25 53.41,9.75 63.91,7.36 128.41,15.75 128.12,5.86 124.52,1.05 128.41,40.95 128.12,47.86 123.61,52.36
  pour Top (isolate 0.406, rank 6): 32.81,53.86 129.81,53.86 129.81,-0.14 41.31,-0.14 41.31,3.44 arc-45 41.61,4.15 42.02,4.56 arc-45 42.73,4.86 46.81,4.86 47.31,5.36 47.31,22.36 48.91,23.56 96.11,23.56 97.61,25.06 97.61,39.95 96.22,40.16 92.91,40.16 88.72,39.95 84.31,40.06 48.71,39.45 47.71,40.45 45.02,42.45 44.52,42.95 40.12,43.86 37.12,46.86 33.81,48.36 32.31,49.86 32.31,53.36
  pour Top (isolate 0.406, no thermals): 48.61,21.15 53.11,21.15 53.11,25.06 47.71,25.06 47.71,21.15
  pour Top (isolate 0.305, no thermals): 81.91,41.56 81.91,44.86 78.92,44.86 78.92,41.56
  pour Top (isolate 0.406, no thermals): 72.61,44.25 74.72,44.25 74.72,41.25 72.61,41.25
  pour Top (isolate 0.305, no thermals): 55.52,15.46 58.21,15.46 58.21,13.36 55.52,13.36
  pour Bottom (isolate 0.406): 39.91,-6.84 40.41,4.66 45.31,8.55 45.91,24.46 79.81,23.65 87.22,20.15 95.02,21.86 94.72,39.66 73.52,39.45 48.41,39.56 36.71,46.66 31.41,49.95 31.41,58.36 136.22,58.36 135.91,-7.04
GND_ISO_RS232  (via drill 0.51, 0.6)
  Top 0.406: U1.15 38.19,14.08 C3.2 C2.2 C1.2 33.13,14.28 C7.2 28.68,14.28 v28.06,13.66 | U1.9 U1.10 31.34,20.43 30.91,20.86 30.91,23.56 28.52,25.96 20.41,25.96 19.38,27 JP1.1 8.39,27.39 DIN1.7 DIN1.8 | DSUB1.5 25.61,11.12 U2.15 25.61,16.41 25.52,16.5 25.52,17.71 25.26,17.96 C10.2
  Bottom 0.406: JP1.1 16.8,27 15.16,25.36 15.16,21.15 16.36,19.96 16.36,15.8 18.91,13.25 20.91,13.25 21.61,12.55 21.61,11 DSUB1.5 25.29,10.8 27.16,10.8 28.06,11.71 v28.06,13.66
  other vias: 38.12,22.06 35.41,22.06 36.91,20.56 40.21,10.96 35.12,9.46 31.81,13.66 33.31,20.86 19.81,15.75 6.31,32.86 9.81,32.86 1.31,29.36 1.31,22.86 1.31,16.86 1.31,10.36 1.81,1.36 9.31,1.36 26.31,1.36 32.81,1.36 32.81,4.36
  pour Top (isolate 0.406): 34.52,-0.45 37.52,4.96 37.81,5.25 42.31,9.16 42.31,21.96 arc90 41.31,22.96 33.31,22.96 29.31,26.76 arc45 28.6,27.06 20.91,27.46 18.91,30.15 12.91,33.16 12.02,33.16 11.41,33.45 10.21,34.66 -1.49,34.66 -1.49,-0.74 -1.19,-0.45
  pour Top (isolate 0.406, no thermals): 41.12,20.25 41.12,24.46 33.62,24.46 33.62,20.25
  pour Bottom (isolate 0.406): -7.19,33.45 -7.49,36.45 10.91,35.36 27.82,26.36 arc25 31.24,24.94 41.52,24.56 44.02,22.36 43.41,9.36 37.71,4.66 36.91,-4.04 -2.38,-2.54 -6.88,33.16
GND_ISO_TRIG  (via drill 0.51)
  Top 0.406: C26.2 C25.2 C24.2 81.79,31.58 U3.15 81.91,33.68 81.91,34.36 | 69.14,31.23 C16.2 | 74.17,34.71 U3.9 74.17,31.16 C28.2 | 74.17,34.71 74.72,35.25 81.02,35.25 81.91,34.36 | U5.9 49.87,35.01 50.11,35.25 57.02,35.25 57.49,34.78 | U5.10 U5.9 | U4.10 U4.9 61.52,33.61 61.52,34.71 | 74.17,34.71 73.62,35.25 69.61,35.25 69.19,34.83 | 57.49,34.78 57.96,35.25 60.91,35.25 61.46,34.71 61.52,34.71 | 61.52,34.71 61.57,34.71 62.11,35.25 68.72,35.25 69.14,34.83 69.19,34.83 | 69.19,34.83 U4.15 69.14,33.51 69.14,31.33 C16.2 | 57.49,34.78 U5.15 57.49,31.43 C29.2 C30.2 | 81.91,34.36 82.81,35.25 83.41,35.25 84.31,34.36 84.31,32.86 85.52,31.65 v85.81,31.65 88.67,31.65 JP2.1 | C16.2 C17.2 | 38.27,31.56 v29.41,31.56 | JP5.10 JP5.9 | 38.35,31.64 38.27,31.56 | 38.27,31.56 49.52,31.56 49.87,31.91 U5.9
  Bottom 0.406: DSUB3.9 11.46,44.21 13.31,42.36 18.11,42.36 27.02,33.45 27.02,32.86 28.31,31.56 v29.41,31.56
  other vias: 84.91,33.45 72.31,34.36 72.92,33.16 48.02,34.36 48.02,32.25 45.62,33.16 60.31,33.45 67.52,29.56 66.61,28.06 85.52,27.46 30.91,42.75 27.62,52.36 23.71,52.36 17.11,52.36 9.31,52.36 4.81,52.36 1.21,52.36 1.21,49.36 8.41,43.36 5.71,43.36
  pour Top (isolate 0.406): 24.31,54.76 30.62,55.06 30.62,51.16 33.91,45.75 33.31,42.75 37.21,42.45 40.81,42.75 47.12,36.75 90.66,36.16 arc-44 91.1,35.97 91.63,35.44 arc-45 91.81,34.99 92.52,26.72 arc-45 92.73,25.87 91,24.14 arc-45 89.55,24.36 82.63,24.36 arc-45 80.92,24.15 80.22,24.25 79.02,24.25 76.81,24.56 75.61,25.75 73.31,26.06 40.91,26.06 35.21,25.86 33.31,26.06 28.47,28.22 arc7 27.06,28.38 20.71,30.15 15.12,36.16 -2.69,38.56 -2.99,42.16 -2.99,54.45 -2.69,54.76
  pour Top (isolate 0.406, no thermals): 79.81,35.56 82.22,35.56 82.22,31.96 79.81,31.96
  pour Top (isolate 0.406, no thermals): 75.02,35.86 75.02,32.56 72.61,32.56 72.61,35.86
  pour Bottom (isolate 0.305): 0.01,53.86 30.52,53.66 30.41,49.16 38.62,44.06 44.12,40.95 49.52,37.95 93.81,38.06 93.61,23.65 86.02,23.86 78.11,25.25 36.15,26.26 arc-26 31.71,27.25 9.21,38.06 -0.19,38.36
IND_EX_1
  Top 0.406: U5.4 54.95,47.22 53.27,48.91 52.21,48.91 51.91,49.2 51.91,51.03 ARD1.10
IND_EX_1_ISO  (via drill 0.51)
  Top 0.406: v38.52,28.61 52.61,28.61 54.95,30.94 U5.13
  Bottom 0.406: DSUB3.6 19.69,43.18 25.52,37.36 29.12,37.36 29.41,37.06 29.41,34.66 30.47,33.6 JP5.3 30.73,32.73 32.21,31.25 37.41,31.25 38.02,30.65 38.02,29.11 v38.52,28.61
IND_EX_2
  Top 0.406: U5.5 53.68,46.24 51.77,48.16 51.02,48.91 49.81,48.91 49.34,49.38 ARD1.11
IND_EX_2_ISO
  Top 0.406: DSUB3.7 16.95,43.82 26.41,34.36 | 26.41,34.36 JP5.2 | 26.41,34.36 26.41,32.56 28.41,30.56 29.71,30.56 30.71,29.56 52.21,29.56 53.68,31.02 U5.12
IND_EX_3
  Top 0.406: 52.52,43.06 U5.6 52.41,46.16 50.56,48 47.71,48 46.81,48.91 ARD1.12
IND_EX_3_ISO  (via drill 0.51)
  Top 0.406: v31.37,30.56 51.77,30.56 52.41,31.2 U5.11
  Bottom 0.406: DSUB3.8 14.2,44.17 15.31,43.06 18.61,43.06 28.07,33.6 JP5.1 | JP5.1 28.21,33.58 | JP5.1 28.2,33.47 28.99,33.47 31.37,31.11 v31.37,30.56
IND_FREQ
  Top 0.406: U5.3 56.22,43.85 55.81,44.25 55.81,47.56 54.42,48.95 ARD1.9
IND_FREQ_ISO  (via drill 0.51)
  Top 0.406: 10.06,44.78 DSUB3.5 10.09,44.08 11.11,43.06 16.52,43.06 25.71,33.86 25.71,32.25 28.12,29.86 29.31,29.86 30.31,28.86 36.41,28.86 37.62,27.65 v40.77,27.65 53.11,27.65 56.27,30.81 56.27,33.31 56.22,33.35 U5.14
  Bottom 0.406: JP5.4 30.73,35.44 32.02,34.16 32.02,32.66 32.71,31.96 38.81,31.96 39.41,31.36 39.41,29.11 v40.77,27.65
IND_START
  Top 0.406: U4.5 65.38,49.32 65.86,49.81 ARD1.5
IND_START_ISO  (via drill 0.51, 0.6)
  Top 0.406: U4.12 65.38,32.52 64.52,31.65 64.52,30.96 63.96,30.4 v63.16,30.4 | JP5.6 33.9,36.14 34.52,36.75 v34.52,40.41
  Bottom 0.406: DSUB3.3 15.62,44.84 15.62,48.45 17.41,50.11 20.41,50.11 23.56,46.95 23.56,42.91 26.06,40.41 v34.52,40.41 39.77,40.41 41.87,38.31 41.87,30.9 43.21,29.56 60.77,29.56 61.61,30.4 v63.16,30.4
IND_STIM  (via drill 0.51)
  Top 0.406: R4.1 95.59,19.06 101.41,19.06 101.58,19.21 JP3.1 101.72,19.81 101.41,20.11 v101.41,25.96 | U4.4 66.65,48.24 68.39,49.98 ARD1.4
  Bottom 0.406: ARD1.4 68.39,49.53 68.86,49.06 93.61,49.06 94.52,48.16 96.31,48.16 97.22,47.25 97.81,47.25 102.02,43.06 102.02,26.56 v101.41,25.96
IND_STIM_ISO  (via drill 0.51, 0.6)
  Top 0.406: U4.13 66.65,32.14 65.27,30.75 65.27,29.86 64.47,29.06 v63.16,29.06 | JP5.7 36.06,33.6 37.12,34.66 v37.12,39.41
  Bottom 0.406: DSUB3.2 18.31,48.31 19.36,49.36 20.11,49.36 22.52,46.95 22.52,42.75 25.87,39.41 v37.12,39.41 39.31,39.41 40.96,37.75 40.96,37.66 40.96,37.16 40.96,30.46 42.77,28.65 61.21,28.65 61.61,29.06 v63.16,29.06
IND_STOP
  Top 0.406: U4.6 64.11,48.56 63.31,49.36 ARD1.6
IND_STOP_ISO  (via drill 0.51, 0.6)
  Top 0.406: U4.11 64.11,32.45 v63.16,31.75 | JP5.5 31.96,34.91 v31.96,41.41
  Bottom 0.406: DSUB3.4 12.91,44.88 12.91,48.75 15.01,50.86 20.71,50.86 24.62,46.95 24.62,43.2 26.41,41.41 v31.96,41.41 40.21,41.41 42.77,38.86 42.77,31.36 43.66,30.46 60.31,30.46 61.36,31.75 v63.16,31.75
IND_SWITCH
  Top 0.406: U4.3 67.92,47.85 69.12,49.06 70.52,49.06 70.94,49.47 ARD1.3
IND_SWITCH_ISO  (via drill 0.6)
  Top 0.406: U4.14 67.92,32.66 67.36,32.11 67.36,31.81 66.17,30.61 66.17,29.4 64.47,27.71 v63.16,27.71
  Bottom 0.406: JP5.8 36.02,36.34 36.02,38.41 | 36.02,38.41 25.66,38.41 21.06,43.01 DSUB3.1 | 36.02,38.41 38.87,38.41 40.06,37.2 40.06,36.86 40.06,30 42.31,27.75 v63.16,27.71
N$1
  Top 0.406: R4.2 95.54,17.21 Q2.B 97.38,14.5 R5.2
N$3
  Top 0.406: Q3.1 R6.2 92.05,10.39 92.37,10.39 92.37,10.91 93.11,11.66 93.95,11.66 Q2.C 94.59,11.81
N$4
  Top 0.406: DSUB1.7 DSUB1.8
N$5
  Top 0.406: Q1.1 84.2,6.39 R1.1 R2.2
N$22
  Top 0.406: U2.1 26.8,20.2 27.8,21.2 27.8,22.15 C8.2
N$23
  Top 0.406: C8.1 25.57,22.46 24.94,21.83 24.94,20.22 U2.3
N$24
  Top 0.406: U2.4 24.31,23.08 C9.2
N$25
  Top 0.406: U2.5 23.66,21.84 23.35,22.15 22.08,22.15 21.76,22.46 C9.1
N$26
  Top 0.406: U2.2 25.61,18.93 25.89,18.65 27.48,18.65 C11.2
N$27
  Top 0.406: U2.6 23.02,21.1 22.66,21.46 20.56,21.46 20.27,21.15 20.27,20.04 C10.1
POT_IN
  Top 0.406: R3.2 90.16,18.82 | 90.16,18.82 90.08,18.82 89.72,18.46 | IC2.1 71.38,16.95 IC1.1 79.89,18.47 81.59,18.47 81.61,18.46 89.8,18.46 90.16,18.82
PWR_STIM
  Top 0.406: R1.2 89.8,5.78 90.61,4.96 105.31,4.96 106.52,6.16 106.52,9.16 107.41,10.05 108.67,10.05 ARD1.52
RESET
  Top 0.406: ARD1.37 119.13,30.74 120.16,29.71 123.27,29.71 DSUB2.8
RS232_RXD
  Top 0.406: U2.14 24.95,11.74 23.87,10.66 19.66,10.66 DSUB1.3
RS232_TXD
  Top 0.406: DSUB1.2 17.51,11.41 23.41,11.41 24.31,12.16 U2.13
SCL  (via drill 0.6)
  Top 0.406: v99.91,21.61 99.16,20.86 96.77,20.86 96.31,21.31 89.41,21.31 88.27,20.15 78.72,20.15 76.81,22.06 72.31,22.06 71.34,21.08 IC2.6
  Bottom 0.406: ARD1.SCL 101.41,48.45 105.61,44.25 105.61,24.46 103.31,22.15 100.41,22.15 100.22,21.96 100.22,21.9 v99.91,21.61
SCLK
  Top 0.406: ARD1.43 118.43,23.11 DSUB2.2
SDA  (via drill 0.6)
  Top 0.406: v99.31,22.96 98.11,21.61 97.22,21.61 96.77,22.06 89.11,22.06 87.91,20.86 79.52,20.86 77.56,22.81 71.92,22.81 70.84,21.73 IC2.7
  Bottom 0.406: v99.31,22.96 102.61,22.96 104.72,25.06 104.72,43.95 98.88,49.8 ARD1.SDA
STIM_OUT
  Top 0.406: J1.1 100.77,9.12 R7.2 Q3.3
  Bottom 0.406: J1.1 101.58,6.59 102.31,5.86 108.27,5.86 110.91,5.86 111.81,5.86 112.61,5.05 112.61,3.55 113.22,2.96 116.36,2.96 116.52,3.11 116.52,4.88 J2.1
STIM_REG_VIN-
  Top 0.406: Q1.3 V1.1 69.3,7.05 C18.1 C14.2
SYNC
  Top 0.406: ARD1.35 118.53,33.28 DSUB2.4
TEST_1
  Top 0.406: ARD1.33 118.73,35.81 DSUB2.5
TEST_2
  Top 0.406: ARD1.45 118.63,20.57 DSUB2.1
TRIG_DISABLE
  Top 0.406: ARD1.7 60.77,49.34 61.21,48.91 62.27,48.91 62.86,48.31 62.86,42.98 U4.7
TRIG_DISABLE_2
  Top 0.406: ARD1.13 44.27,48.75 45.77,47.25 49.96,47.25 51.16,46.06 51.16,42.98 U5.7
TTL_RX  (via drill 0.6)
  Top 0.406: U1.5 51.5,17.89 v51.61,18
  Bottom 0.406: v51.61,18 51.91,18.3 73.52,18.3 76.67,21.46 79.66,21.46 84.31,16.8 95.27,16.8 97.22,18.75 97.22,22.96 98.27,24 102.47,24 103.81,25.36 103.81,43.66 98.66,48.81 97.47,48.81 96.33,49.94 ARD1.RX1
TTL_RX_ISO  (via drill 0.6)
  Top 0.406: v23.87,16.8 23.87,15.75 23.66,15.55 U2.12 | U1.12 37.93,17.89 v37.81,18
  Bottom 0.406: v23.87,16.8 24.02,16.96 27.16,16.96 27.46,17.25 28.96,17.25 30.16,18.46 35.27,18.46 35.71,18 v37.81,18
TTL_TX  (via drill 0.6)
  Top 0.406: U1.3 54.96,15.35 55.66,16.05 55.66,18.75 56.11,19.21 v56.31,19.31
  Bottom 0.406: ARD1.TX1 93.8,50.08 94.81,49.06 96.31,49.06 97.22,48.16 98.11,48.16 102.91,43.36 102.91,25.5 102.31,24.9 97.97,24.9 96.31,23.25 96.31,18.9 94.97,17.55 84.61,17.55 79.97,22.21 76.06,22.21 72.92,19.06 56.56,19.06 v56.31,19.31
TTL_TX_ISO  (via drill 0.6)
  Top 0.406: U1.14 39.52,15.35 39.12,15.75 34.21,15.75 v33.31,16.66 | v22.66,12.46 22.66,13.21 22.96,13.5 22.96,14.51 U2.11
  Bottom 0.406: v33.31,16.66 30.77,16.66 28.96,14.86 27.77,14.86 26.41,13.5 26.41,12.61 25.52,11.71 23.41,11.71 v22.66,12.46
V_ISO_RS232
  Top 0.406: U1.16 40.17,12.56 39.77,12.16 38.21,12.16 C3.1 C2.1 C1.1 33.06,12.3 27.02,12.3 26.27,13.05 U2.16 27.16,14.55 27.8,15.18 C11.1 27.84,16.18 C7.1
V_ISO_TRIG
  Top 0.406: C26.1 C25.1 C24.1 83.06,31.16 U3.16 | U3.10 75.44,32.73 75.92,32.25 75.92,31.11 C28.1 75.92,31 75.92,29.71 | C26.1 83.16,25.4 82.81,25.06 80.41,25.06 79.81,25.65 79.81,28.65 79.22,29.25 76.52,29.25 76.06,29.71 75.92,29.71 | JP2.3 87.02,26.71 86.25,26.25 C26.1 | U5.16 58.76,33.06 59.56,32.25 59.56,31.25 C29.1 C30.1 59.61,27.11 60.02,26.71 70.52,26.71 71.11,27.31 71.11,28.9 C17.1 | C17.1 C16.1 71.17,31.75 70.52,32.41 70.52,33.5 U4.16 | 75.92,29.71 75.61,29.4 71.61,29.4 C17.1
V_SELECT  (via drill 0.6)
  Top 0.406: JP2.2 v85.52,29.25 | v79.22,30.46 79.25,30.49 U3.13
  Bottom 0.406: v79.22,30.46 84.31,30.46 v85.52,29.25
V_STIM
  Top 0.406: Q3.2 R6.1 90.61,8.16 90.31,8.46 90.31,9.86 89.72,10.46 89.72,10.49 88.31,11.89 87.38,12.82 IC1.4 90.46,14.66 C27.2 R3.1
V_STIM_REF
  Top 0.406: C21.1 C23.2 | C23.2 74.38,14.34 V1.4 77.31,14.66 78.31,13.66 78.31,12.43 IC1.3 78.39,12.39 79.52,11.25 79.52,10.18 C22.2 | C34.2 C31.1 73.36,20.4 72.31,20.4 71.69,19.78 IC2.4 69.44,19.78 69.02,19.36 69.02,14.38 C23.2
(copper drawn outside any net)
  shapes: Bottom area x1070

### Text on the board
Bottom: JIMMY 2015
tPlace: SERIAL | I2C | 5V | 5V | GND | Tx | Rx | SDA | SCL | Pmark / in | SWITCH / NETWORK | CS / Extra | ActiChamp / Triggers | Ex_2 | Freq | Start | Switch | GND | UCL EIT / SCOUSETOM / V2.5 | Tst1 | Tst1 | IND | Sync | Ex_3 | Ex_1 | Stop | Stim | GND | 3.3V | Phase MK / for stim | Reset | SEL. IND V | Gnd | DIN+ | GND | 5V | DIN- | PMRK | SCLK | ??? | STIM / (3.3V) | Gnd | Tst2 | TX | RX | RX | BONUS PINS | TX | TX | pmk | Keithley / CS COMM | T | STIM / OUT | R | GND | GND | GND | STIM / OUT | BYLAD | 3v3 | 5V | GND | GND | STIM | Gnd | Gnd | STIM
bPlace: TX | RX

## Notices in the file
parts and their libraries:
SparkFun-DiscreteSemi: Licensing: Creative Commons ShareAlike 4.0 International - https://creativecommons.org/licenses/by-sa/4.0
